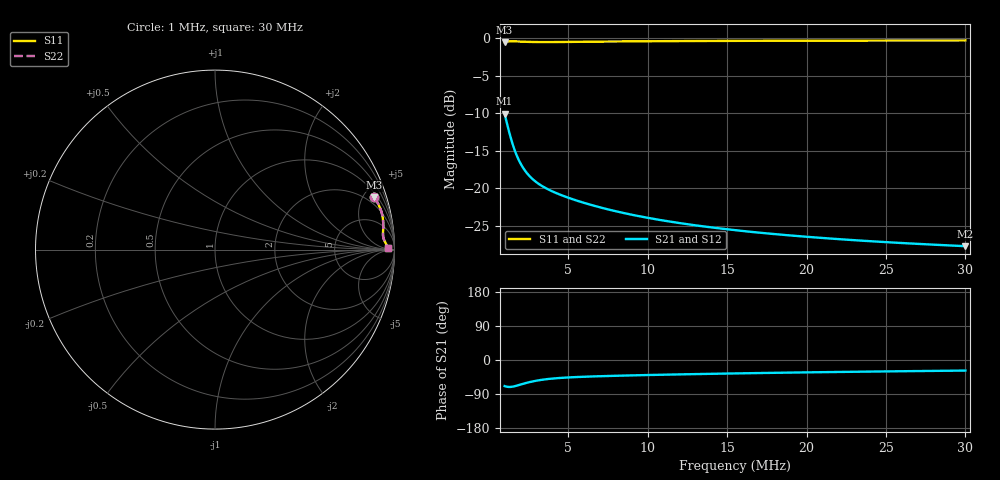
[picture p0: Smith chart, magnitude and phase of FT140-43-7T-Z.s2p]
! ListType=Log
!!BN140-43 7T #20
# MHZ S RI R 50
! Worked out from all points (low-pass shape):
!   101 points, 1 MHz to 30 MHz, reference 50 ohm
!   highest |S21| = -10.05 dB at 1 MHz (marker M1); lowest = -27.7 dB at 30 MHz (marker M2)
!   |S21| within 3 dB of the highest: start of sweep to 1.357 MHz
!   lowest |S11| = -0.6 dB at 1 MHz (marker M3), VSWR 29.00, Z = 65.5 + j297 ohm
!   |S11| at or under -10 dB: nowhere
!   |S22| runs from -0.6 to -0.3 dB; largest |S21 - S12| = 0.00015
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1  0.8864 0.2923  0.1134 -0.2931  0.1134 -0.2932  0.8864 0.2925
1.185376  0.9136 0.2455  0.086 -0.2462  0.0859 -0.2463  0.9137 0.2455
1.405116  0.9298 0.201  0.0699 -0.2017  0.0698 -0.2018  0.9299 0.201
1.556058  0.9345 0.1772  0.0651 -0.178  0.0651 -0.178  0.9346 0.1772
1.723215  0.9367 0.1564  0.063 -0.1573  0.0629 -0.1573  0.9368 0.1565
1.908328  0.9373 0.1389  0.0623 -0.1398  0.0623 -0.1397  0.9373 0.1388
2.113327  0.9372 0.124  0.0624 -0.1249  0.0624 -0.1249  0.9372 0.124
2.262086  0.937 0.1153  0.0627 -0.1164  0.0626 -0.1163  0.937 0.1153
2.505087  0.9365 0.1041  0.0631 -0.1052  0.0631 -0.1052  0.9365 0.1041
2.774191  0.9362 0.0946  0.0635 -0.0958  0.0634 -0.0957  0.9362 0.0946
3.072204  0.936 0.0865  0.0636 -0.0878  0.0636 -0.0878  0.936 0.0865
3.767708  0.9366 0.0737  0.063 -0.0752  0.063 -0.0752  0.9367 0.0737
4.620666  0.9385 0.0638  0.0611 -0.0656  0.0611 -0.0656  0.9386 0.0638
5.862773  0.9419 0.0543  0.0578 -0.0566  0.0578 -0.0566  0.9419 0.0543
6.949589  0.9446 0.0483  0.055 -0.0511  0.055 -0.0511  0.9446 0.0483
8.237875  0.9475 0.0427  0.0521 -0.046  0.0521 -0.046  0.9475 0.0428
10.81396  0.9518 0.0345  0.0478 -0.0387  0.0478 -0.0387  0.9518 0.0345
13.2621  0.9546 0.0287  0.0449 -0.0339  0.0449 -0.0339  0.9546 0.0288
15.72057  0.9566 0.0241  0.0428 -0.0303  0.0428 -0.0303  0.9567 0.0242
20.63659  0.9597 0.0173  0.0398 -0.0252  0.0398 -0.0252  0.9597 0.0173
25.30843  0.9615 0.0122  0.0379 -0.0218  0.0379 -0.0218  0.9616 0.0122
30  0.9629 0.00802  0.0364 -0.0193  0.0365 -0.0193  0.963 0.00805
